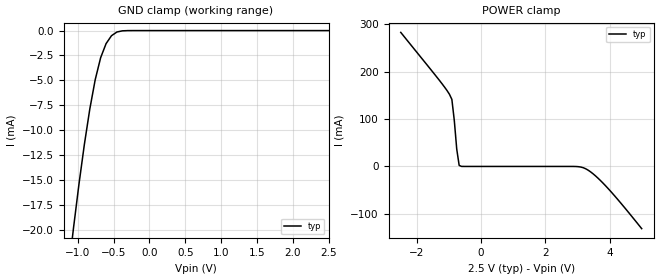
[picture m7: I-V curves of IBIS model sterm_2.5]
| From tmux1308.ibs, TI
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| sterm_2.5
[Model]   sterm_2.5
Model_type   Terminator
|   typ   min   max
C_comp   1.008417e-12   NA   NA
[Voltage Range]   2.5   NA   NA
[Temperature Range]   27   NA   NA
[Power Clamp Reference]   2.5   NA   NA
[GND Clamp Reference]   0   NA   NA
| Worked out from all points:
|   GND clamp passes 1 mA (typ) near -0.58 V on its own axis
|   POWER clamp passes 1 mA (typ) near -0.64 V on its own axis
[GND Clamp]
|   Voltage   I(typ)   I(min)   I(max)
-5V       -20.06kA   NA         NA
-1.136V   -24.52mA   NA         NA
-1.061V   -19.83mA   NA         NA
-909.1mV  -11.44mA   NA         NA
-833.3mV  -7.892mA   NA         NA
-757.6mV  -4.932mA   NA         NA
-681.8mV  -2.725mA   NA         NA
-606.1mV  -1.312mA   NA         NA
-530.3mV  -514.9uA   NA         NA
-454.5mV  -143.4uA   NA         NA
-303mV    -3.396uA   NA         NA
2.5V      1.169nA    NA         NA
[POWER Clamp]
|   Voltage   I(typ)   I(min)   I(max)
-2.5V     282.7mA    NA         NA
-1.212V   174.1mA    NA         NA
-984.9mV  152.3mA    NA         NA
-909.1mV  141.4mA    NA         NA
-833.3mV  96.85mA    NA         NA
-757.6mV  36.5mA     NA         NA
-681.8mV  2.115mA    NA         NA
2.879V    -26.17uA   NA         NA
3.182V    -2.725mA   NA         NA
3.485V    -15.45mA   NA         NA
3.864V    -39.96mA   NA         NA
5V        -131.2mA   NA         NA
